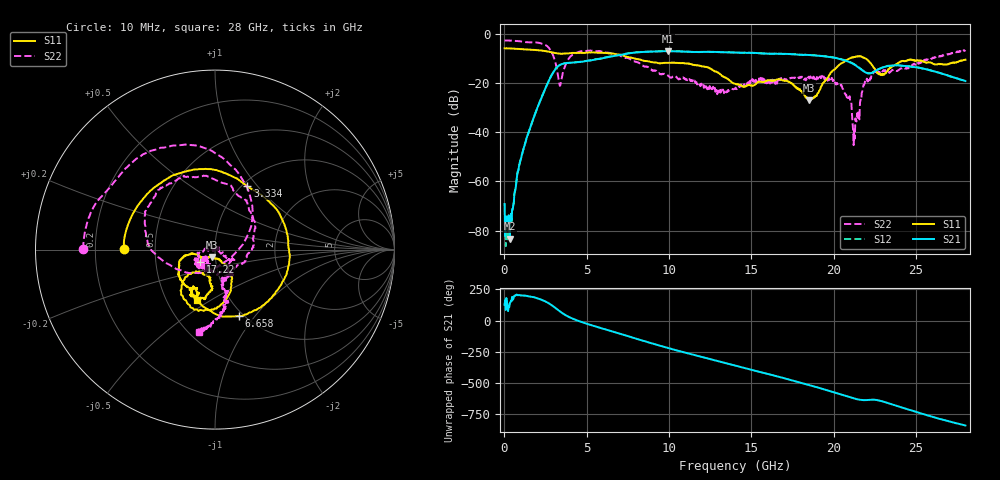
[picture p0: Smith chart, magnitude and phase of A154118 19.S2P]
!  2-Port S-parameters saved by WinCal
! VAR MeasName=S-Parameters (CALIBRATED_DATA) read from VNA (N5230A)
! VAR MeasDate=2015-9-10 14:35:52
! VAR NAME=A154118 19
! VAR FILENAME=A154118 19.S2P
! VAR DATE=2015-9-10 14:35:52
! VAR PHYS_PORTS=1,2
# Hz S DB R 50
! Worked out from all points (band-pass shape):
!   801 points, 10 MHz to 28 GHz, reference 50 ohm
!   highest |S21| = -7.00 dB at 9.911 GHz (marker M1); lowest = -83.3 dB at 324.9 MHz (marker M2)
!   |S21| within 3 dB of the highest: 5.895 GHz to 20.26 GHz (14.36 GHz wide, 110 % of centre)
!   lowest |S11| = -27.0 dB at 18.52 GHz (marker M3), VSWR 1.09, Z = 48.1 - j3.98 ohm
!   |S11| at or under -10 dB: 7.913 GHz to 20.96 GHz (13.04 GHz wide, 90.4 % of centre); 21.91 GHz to end of sweep
!   |S22| runs from -45.3 to -2.7 dB; largest |S21 - S12| = 0.0078
!   S11 on the Smith chart (normalised r, x): 10 MHz: 0.33, +0.00; 3.334 GHz: 1.06, +0.89; 6.658 GHz: 0.95, -0.84; 17.22 GHz: 0.84, -0.12; 28 GHz: 0.71, -0.44
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1e7  -5.89 179.5  -69.21 127.5  -78.08 -116.7  -2.67 179.8
3.248875e8  -5.90 168.6  -83.33 138.0  -79.70 141.8  -2.72 172.1
8.497e8  -6.09 151.1  -55.52 -157.0  -55.39 -155.5  -2.94 158.9
1.374512e9  -6.31 134.0  -41.85 -162.5  -41.87 -162.7  -3.39 146.9
2.5291e9  -7.01 91.4  -21.52 150.2  -21.50 150.5  -4.66 98.8
3.333812e9  -8.05 62.8  -12.77 76.8  -12.74 76.8  -20.36 -32.6
3.963588e9  -7.89 39.8  -11.75 26.2  -11.74 26.3  -9.58 -175.4
4.698325e9  -7.73 8.1  -11.33 -11.6  -11.31 -11.5  -7.05 149.0
6.657625e9  -8.07 -70.2  -8.98 -90.6  -8.90 -90.7  -8.43 86.4
9.351662e9  -11.91 -122.8  -7.17 163.3  -7.10 163.0  -15.94 -29.2
9.911462e9  -11.76 -126.9  -7.00 142.0  -6.98 141.6  -16.82 -60.0
1.194074e10  -13.04 -154.9  -7.37 71.8  -7.33 71.3  -20.26 -142.5
1.4005e10  -20.30 -162.6  -7.60 1.0  -7.57 0.4  -22.33 -123.2
1.722385e10  -19.30 -140.4  -8.19 -108.9  -8.11 -109.6  -18.11 -129.3
1.851839e10  -26.98 -112.7  -8.62 -155.6  -8.57 -155.9  -18.13 -134.4
1.869332e10  -26.02 -91.8  -8.67 -161.8  -8.68 -162.2  -17.26 -130.3
2.04427e10  -12.08 -69.6  -10.34 129.2  -10.29 128.6  -21.04 -169.3
2.093252e10  -10.09 -84.7  -11.39 109.7  -11.26 108.8  -25.91 165.6
2.124741e10  -9.36 -95.1  -12.41 97.3  -12.38 96.5  -39.31 74.0
2.194716e10  -10.04 -127.0  -15.72 84.2  -15.62 83.0  -19.31 -27.0
2.334666e10  -14.37 -96.4  -13.04 58.5  -12.95 57.4  -15.45 -72.5
2.8e10  -10.52 -109.3  -19.19 -118.3  -19.20 -119.1  -6.55 -101.0
